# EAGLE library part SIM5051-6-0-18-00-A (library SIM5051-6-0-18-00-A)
Memory Card Connectors SIM Card ConnectorHinged Type, 6 Pin, SMT, 1.85mm Profile Source: Datasheet
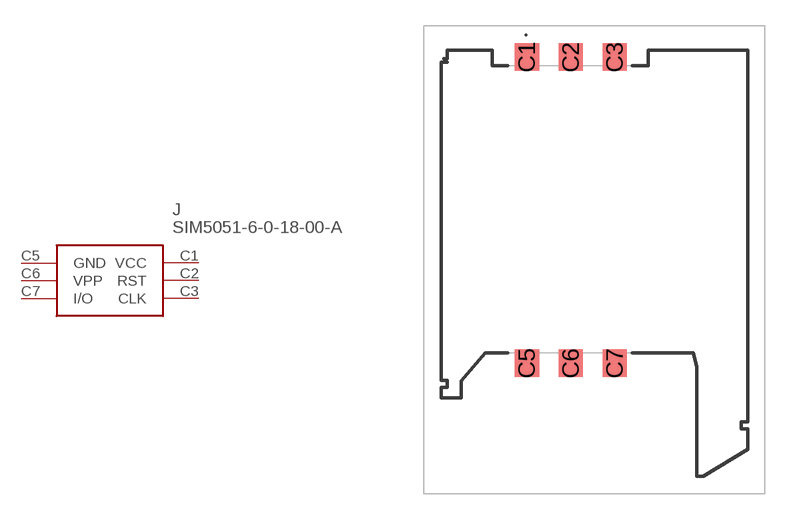
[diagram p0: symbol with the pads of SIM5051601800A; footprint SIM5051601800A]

Designator prefix J

## SIM5051-6-0-18-00-A (Description: Memory Card Connectors SIM Card ConnectorHinged Type, 6 Pin, SMT, 1.85mm Profile; Height: 2mm; Manufacturer_Name: GCT (GLOBAL CONNECTOR TECHNOLOGY); Manufacturer_Part_Number: SIM5051-6-0-18-00-A; Mouser_Part_Number: 640-SIM5051601800A; Mouser_Price-Stock: https://www.mouser.co.uk/ProductDetail/GCT/SIM5051-6-0-18-00-A?qs=KUoIvG%2F9IlalctivsT92PA%3D%3D)  [SIM5051601800A]
C1  VCC
C2  RST
C3  CLK
C5  GND
C6  VPP
C7  I/O

## Footprint SIM5051601800A (pad centres in mm)
SIM5051-6-0-18-00-A-1
smd 1.4 x 1.6: C1 -3.9,11.925; C2 -1.36,11.925; C3 1.18,11.925; C5 -3.9,-5.775; C6 -1.36,-5.775; C7 1.18,-5.775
